FUNCTION_BLOCK FB_IEDClient IMPLEMENTS I_ScsmAbortIndEventSink, I_ScsmGetServerDirectoryCnfEventSink, I_ScsmGetLogicalDeviceDirectoryCnfEventSink, I_ScsmGetLogicalNodeDirectoryCnfEventSink, I_ScsmGetDataValuesCnfEventSink, I_ScsmSetDataValuesCnfEventSink, I_ScsmReportIndEventSink, I_ScsmControlCnfEventSink, I_ScsmLastApplErrorIndEventSink, I_ScsmCommandTerminationIndEventSink
VAR_INPUT
	fbConnection		: FB_iec61850ClientClass := (ipAbortInd:=THIS^, ipGetServerDirectoryCnf:=THIS^, ipGetLogicalDeviceDirectoryCnf:=THIS^, ipGetLogicalNodeDirectoryCnf:=THIS^, ipGetDataValuesCnf:=THIS^, ipSetDataValuesCnf:=THIS^, ipReportInd:=THIS^, ipControlCnf:=THIS^, ipLastApplErrorInd:=THIS^, ipCommandTerminationInd:=THIS^);
END_VAR
VAR
	_bAbort				: BOOL; (* Rising edge activates AbortReq() command execution *)
	_bDisconnect		: BOOL; (* Rising edge activates ReleaseReq() command execution *)
	_bConnect			: BOOL; (* Rising edge activates AssociateReq() command execution *)
	_bReconnect			: BOOL := TRUE; (* TRUE => reconnect automatically *)
	_bReadAllData		: BOOL := TRUE; (* TRUE => read/refresh all data values on reconnect *)
	
	state				: BYTE;
	eState				: E_AsyncEnvironmentState; (* Environment state *)
	bBusy				: BOOL; (* If TRUE => command execution is busy *)
	bSuccess			: BOOL;
	ipResult			: I_AsyncServiceResultClass;
	sLastErrorResult	: T_MaxString;
	fbAbortReason		: FB_ServiceErrorClass := (stError:=SUCCESS_EVENT);
	sLastAbortReason	: T_MaxString;
	nInvokeID			: UDINT;
	eServiceError		: E_AcsiServiceError; (* Latest OnXyzCnf() or OnXyzInd() event handler error *)
	nServiceError		: UDINT; (* Counts OnXyzCnf() and OnXyzInd() event handler errors *)
	nCmdError			: UDINT; (* Counts xyzReq() command errors *)
	sObjReference		: T_AcsiObjectReference; (* DATA object reference *)
	sCtrlReference		: T_AcsiObjectReference; (* CONTROLLABLE-DATA object reference *)
	
	bGetServerDirectory				: BOOL := TRUE; (* Rising edge enumerates logical-devices *)
	bGetLogicalDeviceDirectory		: BOOL := TRUE; (* Rising edge enumerates logical-nodes *)
	bGetLogicalNodeDirectory		: BOOL := TRUE; (* Rising edge enumerates "IEDLD1/LLN0" data-sets *)
	bGetAllServerValues				: BOOL := TRUE; (* Rising edge reads all "IEDLD1" data attribute values *)
	bGetAllDataValues_LLN0_ST		: BOOL := TRUE; (* Rising edge reads all "IEDLD1/LLN0.ST" data attribute values (having selected functional constraint) *)
	bGetDataValues_LLN0_ST_Beh		: BOOL := TRUE; (* Rising edge reads all "IEDLD1/LLN0.ST.Beh" data attribute values (having selected functional constraint) *)
	
	eControl_LLN0_Mod				: E_AcsiCtlService:= E_AcsiCtlService.None; (* Select|Operate|Select&Operate|Cancel starts ENC (Mod) control command *)
	eControl_XCBR_Pos 				: E_AcsiCtlService:= E_AcsiCtlService.None; (* Select|Operate|Select&Operate|Cancel starts DPC control command *)
	eControl_CSWI1_Pos				: E_AcsiCtlService:= E_AcsiCtlService.None; (* Select|Operate|Select&Operate|Cancel starts DPC control command *)
	eControl_LEDGGIO1_AnOut1		: E_AcsiCtlService:= E_AcsiCtlService.None; (* Select|Operate|Select&Operate|Cancel starts APC control command *)
	eControl_LEDGGIO1_SPCSO1		: E_AcsiCtlService:= E_AcsiCtlService.None; (* Select|Operate|Select&Operate|Cancel starts SPC control command *)
	eControl_LEDGGIO1_DPCSO1		: E_AcsiCtlService:= E_AcsiCtlService.None; (* Select|Operate|Select&Operate|Cancel starts DPC control command *)
	eControl_LEDGGIO1_ISCSO1		: E_AcsiCtlService:= E_AcsiCtlService.None; (* Select|Operate|Select&Operate|Cancel starts INC control command *)
	eControl_ATCC1_TapChg			: E_AcsiCtlService:= E_AcsiCtlService.None; (* Select|Operate|Select&Operate|Cancel starts BSC control command *)
	eControl_ATCC1_TapPos			: E_AcsiCtlService:= E_AcsiCtlService.None; (* Select|Operate|Select&Operate|Cancel starts ISC control command *)
	eControl_ATCC1_BndCtrChg		: E_AcsiCtlService:= E_AcsiCtlService.None; (* Select|Operate|Select&Operate|Cancel starts BAC control command *)
	eSimulateDirection_ATCC1_TapPos	: E_AcsiTcmd; (* temp var *)
	
	(* control object's control values *)
	LLN0_Mod_Oper_ctlVal			: E_AcsiMod; (* "IEDLD1/LLN0.CO.Mod.Oper.ctlVal", ENC (Mod) *)	
	XCBR1_Pos_Oper_ctlVal			: BOOL; (* "IEDLD1/XCBR1.CO.Pos.Oper.ctlVal", DPC *)
	CSWI1_Pos_Oper_ctlVal			: BOOL; (* "IEDLD1/CSWI1.CO.Pos.Oper.ctlVal", DPC *)
	LEDGGIO1_AnOut1_Oper_ctlVal_f	: REAL; (* "IEDLD1/LEDGGIO1.CO.AnOut1.Oper.ctlVal.f", APC *)	
	LEDGGIO1_SPCSO1_Oper_ctlVal		: BOOL; (* "IEDLD1/LEDGGIO1.CO.SPCSO1.Oper.ctlVal", SPC *)
	LEDGGIO1_DPCSO1_Oper_ctlVal		: BOOL; (* "IEDLD1/LEDGGIO1.CO.DPCSO1.Oper.ctlVal", DPC *)
	LEDGGIO1_ISCSO1_Oper_ctlVal		: DINT; (* "IEDLD1/LEDGGIO1.CO.ISCSO1.Oper.ctlVal", INC *)	
	ATCC1_TapChg_Oper_ctlVal		: E_AcsiTcmd; (* "IEDLD1/ATCC1.CO.TapChg.Oper.ctlVal", BSC *)
	ATCC1_TapPos_Oper_ctlVal		: SINT(-64..63); (* "IEDLD1/ATCC1.CO.TapPos.Oper.ctlVal", ISC *)	
	ATCC1_BndCtrChg_Oper_ctlVal		: E_AcsiTcmd; (* "EDLD1/ATCC1.CO.BndCtrChg.Oper.ctlVal", BAC *)

	fbSBOwControl					: FB_SBOwControl := (operTm:=NULL_TimeStamp, bTest:=FALSE, eCheck:=E_AcsiCheck.NoCheck); (* Example of control function block implementing "SBO control with normal security (operate-once or operate-many)" *)

	(* control object's status information *) 
	LLN0_Mod_stVal					: E_AcsiMod; (* "IEDLD1/LLN0.ST.Mod.stVal", ENC (Mod) *)
	XCBR1_Pos_stVal					: E_AcsiDbpos; (* "IEDLD1/XCBR1.ST.Pos.stVal", DPC *)
	CSWI1_Pos_stVal					: E_AcsiDbpos; (* "IEDLD1/CSWI1.ST.Pos.stVal", DPC *)
	LEDGGIO1_AnOut1_mxVal_f			: REAL; (* "IEDLD1/LEDGGIO1.MX.AnOut1.mxVal.f", APC *)
	LEDGGIO1_SPCSO1_stVal			: BOOL; (* "IEDLD1/LEDGGIO1.ST.SPCSO1.stVal", SPC *)
	LEDGGIO1_DPCSO1_stVal			: E_AcsiDbpos; (* "IEDLD1/LEDGGIO1.ST.DPCSO1.stVal", DPC *)
	LEDGGIO1_ISCSO1_stVal			: DINT; (* "IEDLD1/LEDGGIO1.ST.ISCSO1.stVal", INC *)
	ATCC1_TapChg_valWTr_posVal		: SINT; (* "IEDLD1/ATCC1.ST.TapChg.valWTr.posVal", BSC *)
	ATCC1_TapPos_valWTr_posVal		: SINT; (* "IEDLD1/ATCC1.ST.TapPos.valWTr.posVal", ISC *)
	ATCC1_BndCtrChg_mxVal_f			: REAL; (* "EDLD1/ATCC1.MX.BndCtrChg.mxVal.f", BAC *)
END_VAR

fbConnection.Execute();
eState:= fbConnection.eState;

CASE state OF
	0: (* Initial state *)
		IF _bAbort THEN (* Abort connection => execute AbortReq() command *)
			_bAbort:= FALSE;
			bSuccess:= fbConnection.AbortReq(ipReason:=fbAbortReason, ipSink:=0, ipResult=>ipResult);
			state:= SEL(bSuccess, 100, 1);
		ELSIF eState = E_AsyncEnvironmentState.Idle AND (_bConnect OR _bReconnect) THEN (* Open/establish connection => execute AssociateReq() command *)
			_bConnect:= FALSE;
			bGetAllServerValues:= SEL(_bReadAllData, bGetAllServerValues, TRUE);
			bSuccess:= fbConnection.AssociateReq(ipSink:=0, ipResult=>ipResult);
			state:= SEL(bSuccess, 100, 1);
		ELSIF eState = E_AsyncEnvironmentState.Established AND _bDisconnect THEN (* Close/release connection => execute ReleaseReq() command *)
			_bDisconnect:= FALSE;
			bSuccess:= fbConnection.ReleaseReq(ipSink:=0, ipResult=>ipResult);
			state:= SEL(bSuccess, 100, 1);
		ELSIF eState = E_AsyncEnvironmentState.Established THEN (* Connection established => exchange IED data *)
			state:= 10;
		END_IF
		_bConnect:= FALSE;
		_bDisconnect:= FALSE;
		(*==================================================================================================================================================================*)
	1: (* Wait for AbortReq() or ReleaseReq() or AssociateReq() command completion *)
		IF ipResult <> 0 THEN
			ipResult.Execute();
			IF NOT (bBusy:=ipResult.IsBusy()) THEN
				state:= SEL(ipResult.IsCompleted(), 100(* failed or aborted *), 0(* succeeded *));
			END_IF
		END_IF
		(*==================================================================================================================================================================*)
	10: (* Read/Write IED data *)
		IF bGetServerDirectory THEN (* Example => execute GetServerDirectoryReq() command *)
			bGetServerDirectory:= FALSE;
			bSuccess:= fbConnection.GetServerDirectoryReq(ipServer:=fbIED, eClass:=E_AcsiServerDirectoryClass.LogicalDevice, hUser:=0, ipSink:=0, nInvokeID=>nInvokeID, ipResult=>ipResult);
			state:= SEL(bSuccess, 100, 11);
		ELSIF bGetLogicalDeviceDirectory THEN (* Example => execute GetLogicalDeviceDirectoryReq() command *)
			bGetLogicalDeviceDirectory:= FALSE;
			bSuccess:= fbConnection.GetLogicalDeviceDirectoryReq(ipLogicalDevice:=fbIED.IEDLD1, hUser:=0, ipSink:=0, nInvokeID=>nInvokeID, ipResult=>ipResult);
			state:= SEL(bSuccess, 100, 11);
		ELSIF bGetLogicalNodeDirectory THEN (* Example => execute GetLogicalNodeDirectoryReq() command *)
			bGetLogicalNodeDirectory:= FALSE;
			bSuccess:= fbConnection.GetLogicalNodeDirectoryReq(ipLogicalNode:=fbIED.IEDLD1.LLN0, eClass:=E_AcsiLogicalNodeClass.DataSet, hUser:=0, ipSink:=0, nInvokeID=>nInvokeID, ipResult=>ipResult);
			state:= SEL(bSuccess, 100, 11);
		ELSIF bGetAllServerValues THEN (* Example => execute GetAllServerValues() command *)
			bGetAllServerValues:= FALSE;
			bSuccess:= fbConnection.GetAllServerValuesReq(ipServer:=fbIED, hUser:=0, ipSink:=0, nInvokeID=>nInvokeID, ipResult=>ipResult);
			state:= SEL(bSuccess, 100, 11);
		ELSIF bGetAllDataValues_LLN0_ST THEN (* Example => execute GetAllDataValuesReq() command *)
			bGetAllDataValues_LLN0_ST:= FALSE;
			bSuccess:= fbConnection.GetAllDataValuesReq(ipLogicalNode:=fbIED.IEDLD1.LLN0, eFc:=E_AcsiFc.ST_, hUser:=0, ipSink:=0, nInvokeID=>nInvokeID, ipResult=>ipResult);
			state:= SEL(bSuccess, 100, 11);
		ELSIF bGetDataValues_LLN0_ST_Beh THEN (* Example => execute GetDataValuesReq() command *)
			bGetDataValues_LLN0_ST_Beh:= FALSE;
			bSuccess:= fbConnection.GetDataValuesReq(ipData:=fbIED.IEDLD1.LLN0.Beh, eFc:=E_AcsiFc.ST_, hUser:=0, ipSink:=0, nInvokeID=>nInvokeID, ipResult=>ipResult);
			state:= SEL(bSuccess, 100, 11);
			(*==================================================================================================================================================================*)
		ELSIF eControl_LLN0_Mod <> E_AcsiCtlService.None THEN (* control ENC (Mod)*)
			IF (eControl_LLN0_Mod = E_AcsiCtlService.Select) OR (eControl_LLN0_Mod = E_AcsiCtlService.SelectAndOperate) THEN
				LLN0_Mod_Oper_ctlVal:= SEL(fbIED.IEDLD1.LLN0.Mod_.stVal.eValue = E_AcsiMod.On, E_AcsiMod.On, E_AcsiMod.OnBlocked);
			END_IF
			bSuccess:= fbSBOwControl.ENC_Mod(ipClient:=fbConnection, ipCtrl:=fbIED.IEDLD1.LLN0.Mod_, ctlVal:=LLN0_Mod_Oper_ctlVal, eControl:= eControl_LLN0_Mod, ipResult=>ipResult);
			eControl_LLN0_Mod:= E_AcsiCtlService.None;
			state:= SEL(bSuccess, 100, 11);
			(*==================================================================================================================================================================*)
		ELSIF eControl_XCBR_Pos <> E_AcsiCtlService.None THEN (* control DPC *)
			IF (eControl_XCBR_Pos = E_AcsiCtlService.Select) OR (eControl_XCBR_Pos = E_AcsiCtlService.SelectAndOperate) THEN
				XCBR1_Pos_Oper_ctlVal:= SEL(fbIED.IEDLD1.XCBR1.Pos.stVal.eValue = E_AcsiDbpos.Off, FALSE, TRUE);
			END_IF
			bSuccess:= fbSBOwControl.DPC(ipClient:=fbConnection, ipCtrl:=fbIED.IEDLD1.XCBR1.Pos, ctlVal:=XCBR1_Pos_Oper_ctlVal, eControl:=eControl_XCBR_Pos, ipResult=>ipResult);
			eControl_XCBR_Pos:= E_AcsiCtlService.None;
			state:= SEL(bSuccess, 100, 11);
			(*==================================================================================================================================================================*)
		ELSIF eControl_CSWI1_Pos <> E_AcsiCtlService.None THEN (* control DPC *)
			IF (eControl_CSWI1_Pos = E_AcsiCtlService.Select) OR (eControl_CSWI1_Pos = E_AcsiCtlService.SelectAndOperate) THEN
				CSWI1_Pos_Oper_ctlVal:= SEL(fbIED.IEDLD1.CSWI1.Pos.stVal.eValue = E_AcsiDbpos.Off, FALSE, TRUE);
			END_IF
			bSuccess:= fbSBOwControl.DPC(ipClient:=fbConnection, ipCtrl:=fbIED.IEDLD1.CSWI1.Pos, ctlVal:=CSWI1_Pos_Oper_ctlVal, eControl:=eControl_CSWI1_Pos, ipResult=>ipResult);
			eControl_CSWI1_Pos:= E_AcsiCtlService.None;
			state:= SEL(bSuccess, 100, 11);
			(*==================================================================================================================================================================*)
		ELSIF eControl_LEDGGIO1_AnOut1 <> E_AcsiCtlService.None THEN (* control APC *)
			IF (eControl_LEDGGIO1_AnOut1 = E_AcsiCtlService.Select) OR (eControl_LEDGGIO1_AnOut1 = E_AcsiCtlService.SelectAndOperate) THEN
				LEDGGIO1_AnOut1_Oper_ctlVal_f:= fbIED.IEDLD1.LEDGGIO1.AnOut1.mxVal.fValue + 1.5;
			END_IF
			bSuccess:= fbSBOwControl.APC(ipClient:=fbConnection, ipCtrl:=fbIED.IEDLD1.LEDGGIO1.AnOut1, ctlVal:=LEDGGIO1_AnOut1_Oper_ctlVal_f, eControl:=eControl_LEDGGIO1_AnOut1, ipResult=>ipResult);
			eControl_LEDGGIO1_AnOut1:= E_AcsiCtlService.None;
			state:= SEL(bSuccess, 100, 11);
			(*==================================================================================================================================================================*)
		ELSIF eControl_LEDGGIO1_SPCSO1 <> E_AcsiCtlService.None THEN (* control SPC *)
			IF (eControl_LEDGGIO1_SPCSO1 = E_AcsiCtlService.Select) OR (eControl_LEDGGIO1_SPCSO1 = E_AcsiCtlService.SelectAndOperate) THEN
				LEDGGIO1_SPCSO1_Oper_ctlVal:= SEL(fbIED.IEDLD1.LEDGGIO1.SPCSO1.stVal.bValue, TRUE(* On *), FALSE(* Off *));(* toggle switch *)
			END_IF
			bSuccess:= fbSBOwControl.SPC(ipClient:=fbConnection, ipCtrl:=fbIED.IEDLD1.LEDGGIO1.SPCSO1, ctlVal:=LEDGGIO1_SPCSO1_Oper_ctlVal, eControl:=eControl_LEDGGIO1_SPCSO1, ipResult=>ipResult);
			eControl_LEDGGIO1_SPCSO1:= E_AcsiCtlService.None;
			state:= SEL(bSuccess, 100, 11);
			(*==================================================================================================================================================================*)
		ELSIF eControl_LEDGGIO1_DPCSO1 <> E_AcsiCtlService.None THEN (* control DPC *)
			IF (eControl_LEDGGIO1_DPCSO1 = E_AcsiCtlService.Select) OR (eControl_LEDGGIO1_DPCSO1 = E_AcsiCtlService.SelectAndOperate) THEN
				LEDGGIO1_DPCSO1_Oper_ctlVal:= SEL(fbIED.IEDLD1.LEDGGIO1.DPCSO1.stVal.eValue = E_AcsiDbpos.Off, FALSE(* Off *), TRUE(* On *));(* toggle switch *)
			END_IF
			bSuccess:= fbSBOwControl.DPC(ipClient:=fbConnection, ipCtrl:=fbIED.IEDLD1.LEDGGIO1.DPCSO1, ctlVal:=LEDGGIO1_DPCSO1_Oper_ctlVal, eControl:=eControl_LEDGGIO1_DPCSO1, ipResult=>ipResult);
			eControl_LEDGGIO1_DPCSO1:= E_AcsiCtlService.None;
			state:= SEL(bSuccess, 100, 11);
			(*==================================================================================================================================================================*)
		ELSIF eControl_LEDGGIO1_ISCSO1 <> E_AcsiCtlService.None THEN (* control INC *)
			IF (eControl_LEDGGIO1_ISCSO1 = E_AcsiCtlService.Select) OR (eControl_LEDGGIO1_ISCSO1 = E_AcsiCtlService.SelectAndOperate) THEN
				LEDGGIO1_ISCSO1_Oper_ctlVal:= fbIED.IEDLD1.LEDGGIO1.ISCSO1.stVal.iValue + 1;
			END_IF
			bSuccess:= fbSBOwControl.INC(ipClient:=fbConnection, ipCtrl:=fbIED.IEDLD1.LEDGGIO1.ISCSO1, ctlVal:=LEDGGIO1_ISCSO1_Oper_ctlVal, eControl:=eControl_LEDGGIO1_ISCSO1, ipResult=>ipResult);
			eControl_LEDGGIO1_ISCSO1:= E_AcsiCtlService.None;
			state:= SEL(bSuccess, 100, 11);
			(*==================================================================================================================================================================*)
		ELSIF eControl_ATCC1_TapChg <> E_AcsiCtlService.None THEN (* control BSC *)
			IF (eControl_ATCC1_TapChg = E_AcsiCtlService.Select) OR (eControl_ATCC1_TapChg = E_AcsiCtlService.SelectAndOperate) THEN
				IF fbIED.IEDLD1.ATCC1.TapChg.valWTr.posVal.iValue >= 10 THEN
					ATCC1_TapChg_Oper_ctlVal:= E_AcsiTcmd.Lower;
				ELSIF fbIED.IEDLD1.ATCC1.TapChg.valWTr.posVal.iValue <= -10 THEN
					ATCC1_TapChg_Oper_ctlVal:= E_AcsiTcmd.Higher;
				ELSIF ATCC1_TapChg_Oper_ctlVal = E_AcsiTcmd.Stop THEN
					ATCC1_TapChg_Oper_ctlVal:= E_AcsiTcmd.Higher;
				END_IF
			END_IF
			bSuccess:= fbSBOwControl.BSC(ipClient:=fbConnection, ipCtrl:=fbIED.IEDLD1.ATCC1.TapChg, ctlVal:=ATCC1_TapChg_Oper_ctlVal, eControl:=eControl_ATCC1_TapChg, ipResult=>ipResult);
			eControl_ATCC1_TapChg:= E_AcsiCtlService.None;
			state:= SEL(bSuccess, 100, 11);
			(*==================================================================================================================================================================*)
		ELSIF eControl_ATCC1_TapPos <> E_AcsiCtlService.None THEN (* control ISC *)
			IF (eControl_ATCC1_TapPos = E_AcsiCtlService.Select) OR (eControl_ATCC1_TapPos = E_AcsiCtlService.SelectAndOperate) THEN
				IF fbIED.IEDLD1.ATCC1.TapPos.valWTr.posVal.iValue >= 63 THEN
					eSimulateDirection_ATCC1_TapPos:= E_AcsiTcmd.Lower;
				ELSIF fbIED.IEDLD1.ATCC1.TapPos.valWTr.posVal.iValue <= -64 THEN
					eSimulateDirection_ATCC1_TapPos:= E_AcsiTcmd.Higher;
				ELSIF eSimulateDirection_ATCC1_TapPos = E_AcsiTcmd.Stop THEN
					eSimulateDirection_ATCC1_TapPos:= E_AcsiTcmd.Higher;
				END_IF
				ATCC1_TapPos_Oper_ctlVal:= SEL(eSimulateDirection_ATCC1_TapPos = E_AcsiTcmd.Higher, fbIED.IEDLD1.ATCC1.TapPos.valWTr.posVal.iValue - 1, fbIED.IEDLD1.ATCC1.TapPos.valWTr.posVal.iValue + 1);
			END_IF
			bSuccess:= fbSBOwControl.ISC(ipClient:=fbConnection, ipCtrl:=fbIED.IEDLD1.ATCC1.TapPos, ctlVal:=ATCC1_TapPos_Oper_ctlVal, eControl:=eControl_ATCC1_TapPos, ipResult=>ipResult);
			eControl_ATCC1_TapPos:= E_AcsiCtlService.None;
			state:= SEL(bSuccess, 100, 11);
			(*==================================================================================================================================================================*)
		ELSIF eControl_ATCC1_BndCtrChg <> E_AcsiCtlService.None THEN (* control BAC *)
			IF (eControl_ATCC1_BndCtrChg = E_AcsiCtlService.Select) OR (eControl_ATCC1_BndCtrChg = E_AcsiCtlService.SelectAndOperate) THEN
				IF fbIED.IEDLD1.ATCC1.BndCtrChg.mxVal.f.fValue >= 10.0 THEN
					ATCC1_BndCtrChg_Oper_ctlVal:= E_AcsiTcmd.Lower;
				ELSIF fbIED.IEDLD1.ATCC1.BndCtrChg.mxVal.f.fValue <= -10.0 THEN
					ATCC1_BndCtrChg_Oper_ctlVal:= E_AcsiTcmd.Higher;
				ELSIF ATCC1_BndCtrChg_Oper_ctlVal = E_AcsiTcmd.Stop THEN
					ATCC1_BndCtrChg_Oper_ctlVal:= E_AcsiTcmd.Higher;
				END_IF
			END_IF
			bSuccess:= fbSBOwControl.BAC(ipClient:=fbConnection, ipCtrl:=fbIED.IEDLD1.ATCC1.BndCtrChg, ctlVal:=ATCC1_BndCtrChg_Oper_ctlVal, eControl:=eControl_ATCC1_BndCtrChg, ipResult=>ipResult);
			eControl_ATCC1_BndCtrChg:= E_AcsiCtlService.None;
			state:= SEL(bSuccess, 100, 11);
		ELSE
			state:= 0;
		END_IF
		(*==================================================================================================================================================================*)
	11: (* Wait for GetServerDirectoryReq(), GetLogicalDeviceDirectoryReq(), GetLogicalNodeDirectoryReq(), GetAllServerValuesReq(), GetAllDataValuesReq(), GetDataValuesReq()
		or APC|BAC|BSC|DPC|ENC(Mod)|INC|ISC|SPC control command completion *)
		IF ipResult <> 0 THEN
			ipResult.Execute();
			IF NOT (bBusy:=ipResult.IsBusy()) THEN
				state:= SEL(ipResult.IsCompleted(), 100(* failed or aborted *), 0(* succeeded *));
			END_IF
		END_IF
		(*==================================================================================================================================================================*)
	100: (* Error state *)
		state:= 0;
		IF ipResult <> 0 THEN
			nCmdError:= nCmdError + 1;
			sLastErrorResult:= ipResult.Dump();
			fbSBOwControl.Clear(ipReason:=ipResult.ipError);
		END_IF
END_CASE

LLN0_Mod_stVal:= fbIED.IEDLD1.LLN0.Mod_.stVal.eValue;
XCBR1_Pos_stVal:= fbIED.IEDLD1.XCBR1.Pos.stVal.eValue;
CSWI1_Pos_stVal:= fbIED.IEDLD1.CSWI1.Pos.stVal.eValue;
LEDGGIO1_AnOut1_mxVal_f:= fbIED.IEDLD1.LEDGGIO1.AnOut1.mxVal.f.fValue; 
LEDGGIO1_SPCSO1_stVal:= fbIED.IEDLD1.LEDGGIO1.SPCSO1.stVal.bValue;
LEDGGIO1_DPCSO1_stVal:= fbIED.IEDLD1.LEDGGIO1.DPCSO1.stVal.eValue;
LEDGGIO1_ISCSO1_stVal:= fbIED.IEDLD1.LEDGGIO1.ISCSO1.stVal.iValue;
ATCC1_TapChg_valWTr_posVal:= fbIED.IEDLD1.ATCC1.TapChg.valWTr.posVal.iValue;
ATCC1_TapPos_valWTr_posVal:= fbIED.IEDLD1.ATCC1.TapPos.valWTr.posVal.iValue;
ATCC1_BndCtrChg_mxVal_f:= fbIED.IEDLD1.ATCC1.BndCtrChg.mxVal.f.fValue;

PROPERTY bAbort : BOOL
SET
_bAbort:= bAbort;
END_SET
END_PROPERTY

PROPERTY bConnect : BOOL
SET
_bConnect:= bConnect;
END_SET
END_PROPERTY

PROPERTY bDisconnect : BOOL
SET
_bDisconnect:= bDisconnect;
END_SET
END_PROPERTY

PROPERTY bReconnect : BOOL
SET
_bReconnect:= bReconnect;
END_SET
END_PROPERTY

(* This method receives IEC61850::Abort.ind primitive. *)
METHOD OnAbortInd
VAR_INPUT
	ipAA		: I_ScsmAssociationClass; (* Application association. If = 0 => optional. *)
	bPAbort		: BOOL; (* TRUE => P-Abort.request(), issued by provider, FALSE => Abort.request(), issued by user. *)
	ipReason	: I_ServiceErrorClass; (* Abort reason. *)
	ipData		: I_BaseStreamClass; (* Optional data. If = 0 => default, no data. *)
END_VAR
VAR
END_VAR
IF ipReason <> 0 THEN
	sLastAbortReason:= ipReason.Dump();
END_IF
END_METHOD

(* This method receives buffered IEC61850::Report.ind primitive. *)
METHOD OnBufferedReportInd
VAR_INPUT
	ipAA		: I_ScsmAssociationClass; (* Application association. If = 0 => optional. *)
	info		: ST_ScsmReportEventInfo;
	ipBrcb		: I_AcsiCommonBufferedReportControlBlockClass; (* Interface pointer to BRCB object. *)
	ipDataSet	: I_AcsiCommonDataSetClass; (* Interface pointer to data-set object. *)
	ipData		: I_AcsiCommonDataClass; (* Interface pointer to reported data object. *)
	eFc			: E_AcsiFc; (* Functional constraint of reported data. *)
	eError		: E_AcsiServiceError; (* Data access error code. *)
END_VAR
VAR
END_VAR
IF eError <> E_AcsiServiceError.NoError THEN
	eServiceError:= eError;
	nServiceError:= nServiceError + 1;
END_IF
IF ipData <> 0 THEN
	sObjReference:= ipData.GetObjectReference();
END_IF
END_METHOD

(* This method receives IEC61850::CommandTermination.ind primitive. *)
METHOD OnCommandTerminationInd
VAR_INPUT
	ipAA		: I_ScsmAssociationClass; (* Application association. If = 0 => optional. *)
	info		: ST_ScsmCommandTerminationEventInfo;
	ipCtrl		: I_AcsiCommonControllableDataClass; (* Interface pointer to controllable data object. *)
	ipData		: I_AcsiCommonDataClass; (* Interface pointer to Oper/Cancel/SBO or SBOw data object. *)
	eFc			: E_AcsiFc; (* Functional constraint (CO). *)
	eError		: E_AcsiServiceError; (* Error code. *)
END_VAR
VAR
END_VAR
IF eError <> E_AcsiServiceError.NoError THEN
	eServiceError:= eError;
	nServiceError:= nServiceError + 1;
END_IF
IF ipCtrl <> 0 THEN
	sCtrlReference:= ipCtrl.GetObjectReference();
END_IF
IF ipData <> 0 THEN
	sObjReference:= ipData.GetObjectReference();
END_IF
IF fbSBOwControl.ctlNum = info.CtlNum THEN
	fbSBOwControl.OnCommandTerminationInd( ipCtrl := ipCtrl );
END_IF
END_METHOD

(* This method receives IEC61850::Control[Select|Operate|SelectWithValue|Cancel].cnf primitive. *)
METHOD OnControlCnf
VAR_INPUT
	ipAA		: I_ScsmAssociationClass; (* Application association. If = 0 => optional. *)
	info		: ST_ScsmConfirmedEventInfo;
	ipCtrl		: I_AcsiCommonControllableDataClass; (* Interface pointer to controllable data object. *)
	ipData		: I_AcsiCommonDataClass; (* Interface pointer to Oper/Cancel/SBO or SBOw data object. *)
	eFc			: E_AcsiFc; (* Functional constraint (CO). *)
	eError		: E_AcsiServiceError; (* Write/Read data access error code. *)
END_VAR
VAR
END_VAR
IF eError <> E_AcsiServiceError.NoError THEN
	eServiceError:= eError;
	nServiceError:= nServiceError + 1;
END_IF
IF ipCtrl <> 0 THEN
	sCtrlReference:= ipCtrl.GetObjectReference();
END_IF
IF ipData <> 0 THEN
	sObjReference:= ipData.GetObjectReference();
END_IF
IF NOT info.bMoreFollows THEN
	fbSBOwControl.OnControlCnf( ipCtrl := ipCtrl );
END_IF
END_METHOD

(* This method receives IEC61850::GetDataValues.cnf primitive. *)
METHOD OnGetDataValuesCnf
VAR_INPUT
	ipAA		: I_ScsmAssociationClass; (* Application association. If = 0 => optional. *)
	info		: ST_ScsmConfirmedEventInfo;
	ipData		: I_AcsiCommonDataClass; (* Interface pointer to read data object. *)
	eFc			: E_AcsiFc; (* Functional constraint of read data. *)
	eError		: E_AcsiServiceError; (* Data access error code. *)
END_VAR
VAR
END_VAR
IF eError <> E_AcsiServiceError.NoError THEN
	eServiceError:= eError;
	nServiceError:= nServiceError + 1;
END_IF
IF ipData <> 0 THEN
	sObjReference:= ipData.GetObjectReference();
END_IF
END_METHOD

(* This method receives IEC61850::GetLogicalDeviceDirectory.cnf primitive. *)
METHOD OnGetLogicalDeviceDirectoryCnf
VAR_INPUT
	ipAA				: I_ScsmAssociationClass; (* Application association. If = 0 => optional. *)
	info				: ST_ScsmConfirmedEventInfo;
	ipLogicalDevice		: I_AcsiCommonLogicalDeviceClass; (* Interface pointer to logical-device object. *)
	sObjectReference	: T_AcsiObjectReference;
	eError				: E_AcsiServiceError; (* Logical-device class access error code. *)
END_VAR
VAR
END_VAR
IF eError <> E_AcsiServiceError.NoError THEN
	eServiceError:= eError;
	nServiceError:= nServiceError + 1;
END_IF
sObjReference:= sObjectReference;
END_METHOD

(* This method receives IEC61850::GetLogicalNodeDirectory.cnf primitive. *)
METHOD OnGetLogicalNodeDirectoryCnf
VAR_INPUT
	ipAA				: I_ScsmAssociationClass; (* Application association. If = 0 => optional. *)
	info				: ST_ScsmConfirmedEventInfo;
	ipLogicalNode		: I_AcsiCommonLogicalNodeClass; (* Interface pointer to logical-node object. *)
	eClass				: E_AcsiLogicalNodeClass; (* Logical-node directory class (BRCB, URCB, DATA-SET, ... ). *)
	sObjectReference	: T_AcsiObjectReference;
	eError				: E_AcsiServiceError; (* Logical-node class access error code. *)
END_VAR
VAR
END_VAR
IF eError <> E_AcsiServiceError.NoError THEN
	eServiceError:= eError;
	nServiceError:= nServiceError + 1;
END_IF
sObjReference:= sObjectReference;
END_METHOD

(* This method receives IEC61850::GetServerDirectory.cnf primitive. *)
METHOD OnGetServerDirectoryCnf
VAR_INPUT
	ipAA				: I_ScsmAssociationClass; (* Application association. If = 0 => optional. *)
	info				: ST_ScsmConfirmedEventInfo;
	ipServer			: I_AcsiCommonIntelligentElectronicDeviceClass; (* Interface pointer to server object. *)
	eClass				: E_AcsiServerDirectoryClass; (* Server directory class (logical-device or file). *)
	sObjectReference	: T_AcsiObjectReference;
	eError				: E_AcsiServiceError; (* Server class (logical-device) access error code. *)
END_VAR
VAR
END_VAR
IF eError <> E_AcsiServiceError.NoError THEN
	eServiceError:= eError;
	nServiceError:= nServiceError + 1;
END_IF
sObjReference:= sObjectReference;
END_METHOD

(* This method receives IEC61850::LastApplError.ind primitive. *)
METHOD OnLastApplErrorInd
VAR_INPUT
	ipAA		: I_ScsmAssociationClass; (* Application association. If = 0 => optional. *)
	info		: ST_ScsmAdditionalCauseDiagnosticEventInfo;
	ipCtrl		: I_AcsiCommonControllableDataClass; (* Interface pointer to controllable data object. *)
	eError		: E_AcsiServiceError; (* Error code. *)
END_VAR
VAR
END_VAR
IF eError <> E_AcsiServiceError.NoError THEN
	eServiceError:= eError;
	nServiceError:= nServiceError + 1;
END_IF
IF ipCtrl <> 0 THEN
	sCtrlReference:= ipCtrl.GetObjectReference();
END_IF
IF fbSBOwControl.ctlNum = info.CtlNum THEN
	fbSBOwControl.OnLastApplErrorInd( ipCtrl := ipCtrl );
END_IF
END_METHOD

(* This method receives IEC61850::SetDataValues.cnf primitive. *)
METHOD OnSetDataValuesCnf
VAR_INPUT
	ipAA		: I_ScsmAssociationClass; (* Application association. If = 0 => optional. *)
	info		: ST_ScsmConfirmedEventInfo;
	ipData		: I_AcsiCommonDataClass; (* Interface pointer to written data object. *)
	eFc			: E_AcsiFc; (* Functional constraint of written data. *)
	eError		: E_AcsiServiceError; (* Data access error code. *)
END_VAR
VAR
END_VAR
IF eError <> E_AcsiServiceError.NoError THEN
	eServiceError:= eError;
	nServiceError:= nServiceError + 1;
END_IF
IF ipData <> 0 THEN
	sObjReference:= ipData.GetObjectReference();
END_IF
END_METHOD

(* This method receives unbuffered IEC61850::Report.ind primitive. *)
METHOD OnUnbufferedReportInd
VAR_INPUT
	ipAA		: I_ScsmAssociationClass; (* Application association. If = 0 => optional. *)
	info		: ST_ScsmReportEventInfo;
	ipUrcb		: I_AcsiCommonUnbufferedReportControlBlockClass; (* Interface pointer to URCB object. *)
	ipDataSet	: I_AcsiCommonDataSetClass; (* Interface pointer to dataset object. *)
	ipData		: I_AcsiCommonDataClass; (* Interface pointer to reported data object. *)
	eFc			: E_AcsiFc; (* Functional constraint of reported data. *)
	eError		: E_AcsiServiceError; (* Data access error code. *)
END_VAR
VAR
END_VAR
IF eError <> E_AcsiServiceError.NoError THEN
	eServiceError:= eError;
	nServiceError:= nServiceError + 1;
END_IF
IF ipData <> 0 THEN
	sObjReference:= ipData.GetObjectReference();
END_IF
END_METHOD

END_FUNCTION_BLOCK
